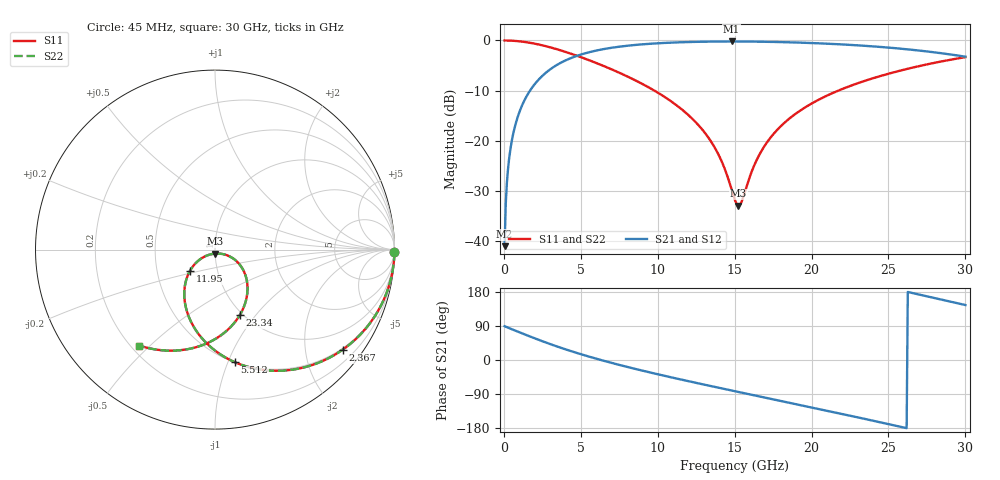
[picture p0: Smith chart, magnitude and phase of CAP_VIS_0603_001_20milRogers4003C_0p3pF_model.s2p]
! S-parameter model data by Modelithics Inc.  support@modelithics.com  813-866-6335  Tampa FL USA
! S-Parameter data specifications:
! Substrate: 20-mil Rogers 4003C, substrate thickness, H=0.508mm, Dielectric constant, Er=3.75
! PCB Mounting Pad Footprint: Pad width, PadW=0.90mm , Pad length, PadL=1.00mm , Pad gap, PadG (edge-to-edge)=1.00mm , Reference planes=3.0mm apart
! Created Wed Nov 18 13:16:05 2015
# hz S ma R 50
! 2 Port Network Data from SP1.SP block
! freq  magS11  angS11  magS21  angS21  magS12  angS12  magS22  angS22
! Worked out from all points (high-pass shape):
!   401 points, 45 MHz to 30 GHz, reference 50 ohm
!   highest |S21| = -0.21 dB at 14.8 GHz (marker M1); lowest = -41.1 dB at 45 MHz (marker M2)
!   |S21| within 3 dB of the highest: 4.624 GHz to 29.92 GHz (25.3 GHz wide, 146 % of centre)
!   lowest |S11| = -33.0 dB at 15.25 GHz (marker M3), VSWR 1.05, Z = 50.1 - j2.23 ohm
!   |S11| at or under -10 dB: 9.769 GHz to 21.76 GHz (11.99 GHz wide, 76 % of centre)
!   |S22| runs from -33.0 to 0.0 dB; largest |S21 - S12| = 0
!   S11 on the Smith chart (normalised r, x): 45 MHz: open; 2.367 GHz: 0.46, -2.82; 5.512 GHz: 0.50, -1.06; 11.95 GHz: 0.74, -0.18; 23.34 GHz: 0.97, -0.83; 30 GHz: 0.23, -0.46
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4.5e7  0.9999 -0.8  0.008811 89.2  0.008811 89.2  0.9999 -0.8
3.4455e8  0.9975 -5.8  0.06708 84.0  0.06708 84.0  0.9975 -5.8
7.189875e8  0.9898 -12.0  0.1388 77.8  0.1388 77.8  0.9898 -12.0
1.392975e9  0.9638 -22.9  0.2628 66.9  0.2628 66.9  0.9638 -22.9
2.366512e9  0.9037 -38.1  0.4234 51.6  0.4234 51.6  0.9037 -38.1
3.6396e9  0.8007 -56.4  0.5923 33.1  0.5923 33.1  0.8007 -56.4
5.062462e9  0.6759 -74.7  0.7279 14.6  0.7279 14.6  0.6759 -74.7
5.511788e9  0.637 -80.0  0.761 9.2  0.761 9.2  0.637 -80.0
7.683525e9  0.4622 -103.3  0.8735 -14.8  0.8735 -14.8  0.4622 -103.3
1.007992e10  0.2961 -125.3  0.9385 -38.4  0.9385 -38.4  0.2961 -125.3
1.195211e10  0.1821 -139.8  0.9641 -55.5  0.9641 -55.5  0.1821 -139.8
1.367452e10  0.08671 -147.1  0.9748 -70.7  0.9748 -70.7  0.08671 -147.1
1.479784e10  0.03265 -128.7  0.9766 -80.5  0.9766 -80.5  0.03265 -128.7
1.50225e10  0.02539 -112.2  0.9765 -82.4  0.9765 -82.4  0.02539 -112.2
1.524716e10  0.02233 -86.8  0.9763 -84.4  0.9763 -84.4  0.02233 -86.8
1.637048e10  0.06107 -26.8  0.9732 -94.0  0.9732 -94.0  0.06107 -26.8
1.719424e10  0.1004 -25.3  0.969 -101.1  0.969 -101.1  0.1004 -25.3
2.003996e10  0.2361 -42.4  0.942 -125.5  0.942 -125.5  0.2361 -42.4
2.333501e10  0.3891 -69.1  0.8869 -154.3  0.8869 -154.3  0.3891 -69.1
2.505742e10  0.4677 -83.9  0.8472 -169.7  0.8472 -169.7  0.4677 -83.9
2.730405e10  0.568 -103.9  0.7832 169.9  0.7832 169.9  0.568 -103.9
3e10  0.6813 -128.4  0.6884 145.0  0.6884 145.0  0.6813 -128.4
